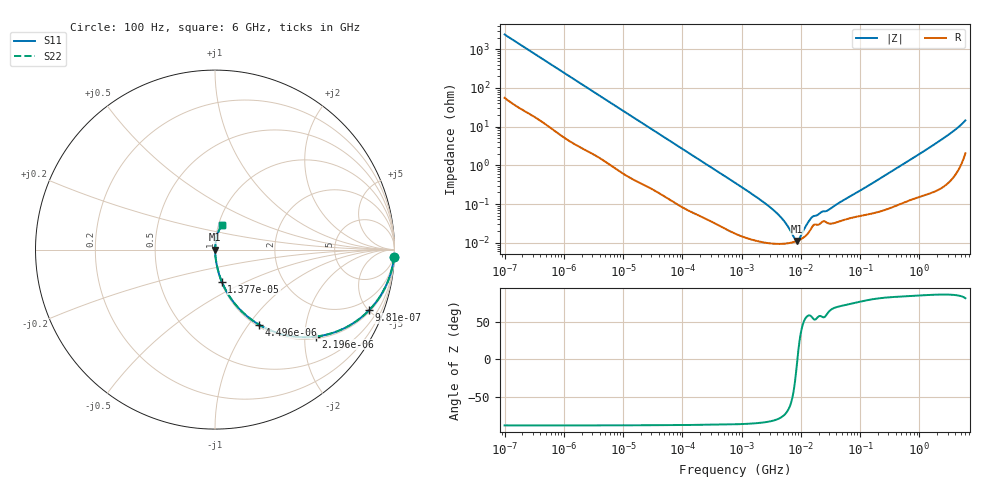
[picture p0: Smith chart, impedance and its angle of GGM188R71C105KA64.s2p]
!Murata Part Number: GGM188R71C105KA64
!These Parameters are Measured in Series Mode Connection
!Data Generated on Mar 13, 2026
!  o--ll--o
!Port1  Port2
!  o------o
!Operation Temp=25[degC], DC Bias Voltage=0[V]
!Freq. Start=100[Hz] Stop=6[GHz] 401[Steps]
# Hz S RI R 50
!Freq.(Hz) S11(Real) S11(Imag) S21(Real) S21(Imag) S12(Real) S12(Imag) S22(Real) S22(Imag)
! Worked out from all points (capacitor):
!   401 points, 100 Hz to 6 GHz, reference 50 ohm
!   read as one part in series: C = 660 nF near 109 Hz
!   lowest |Z| = 11.2 mohm at 8.692 MHz (marker M1)
!   series resonance near 8.764 MHz, so ESL is about 500 pH
!   S11 on the Smith chart (normalised r, x): 100 Hz: 2, -48; 981 Hz: 1.11, -5.05; 2.196 kHz: 1.05, -2.28; 4.496 kHz: 1.03, -1.13; 13.77 kHz: 1.01, -0.37; 6 GHz: 1.04, +0.29
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100  0.9973 -0.0415  0.00268 0.0415  0.00268 0.0415  0.9973 -0.0415
335  0.9785 -0.1339  0.0215 0.1339  0.0215 0.1339  0.9785 -0.1339
981  0.8593 -0.3373  0.1407 0.3373  0.1407 0.3373  0.8593 -0.3373
2008  0.6051 -0.4777  0.3949 0.4777  0.3949 0.4777  0.6051 -0.4777
2196  0.5632 -0.4847  0.4368 0.4847  0.4368 0.4847  0.5632 -0.4847
4496  0.2461 -0.4186  0.7539 0.4186  0.7539 0.4186  0.2461 -0.4186
7358  0.1131 -0.3049  0.8869 0.3049  0.8869 0.3049  0.1131 -0.3049
13772  0.0378 -0.1788  0.9622 0.1788  0.9622 0.1788  0.0378 -0.1788
40335  0.0061 -0.0644  0.9939 0.0644  0.9939 0.0644  0.0061 -0.0644
774597  0.000185 -0.00356  0.9998 0.00356  0.9998 0.00356  0.000185 -0.00356
2074311  0.000108 -0.00128  0.9999 0.00128  0.9999 0.00128  0.000108 -0.00128
3712478  9.45e-05 -0.000628  0.9999 0.000628  0.9999 0.000628  9.45e-05 -0.000628
5311619  9.5e-05 -0.00034  0.9999 0.00034  0.9999 0.00034  9.5e-05 -0.00034
7947587  0.000107 -6.42e-05  0.9999 6.42e-05  0.9999 6.42e-05  0.000107 -6.42e-05
8692127  0.000112 -5.3e-06  0.9999 5.3e-06  0.9999 5.3e-06  0.000112 -5.3e-06
9506416  0.000119 5.39e-05  0.9999 -5.39e-05  0.9999 -5.39e-05  0.000119 5.39e-05
1.300572e7  0.00017 0.000273  0.9998 -0.000273  0.9998 -0.000273  0.00017 0.000273
1.555665e7  0.000258 0.000386  0.9997 -0.000386  0.9997 -0.000386  0.000258 0.000386
2.911731e7  0.000319 0.000624  0.9997 -0.000624  0.9997 -0.000624  0.000319 0.000624
3.124326e8  0.000814 0.00641  0.9992 -0.00641  0.9992 -0.00641  0.000814 0.00641
2.240541e9  0.00434 0.0433  0.9957 -0.0433  0.9957 -0.0433  0.00434 0.0433
6e9  0.0391 0.1353  0.9609 -0.1353  0.9609 -0.1353  0.0391 0.1353
